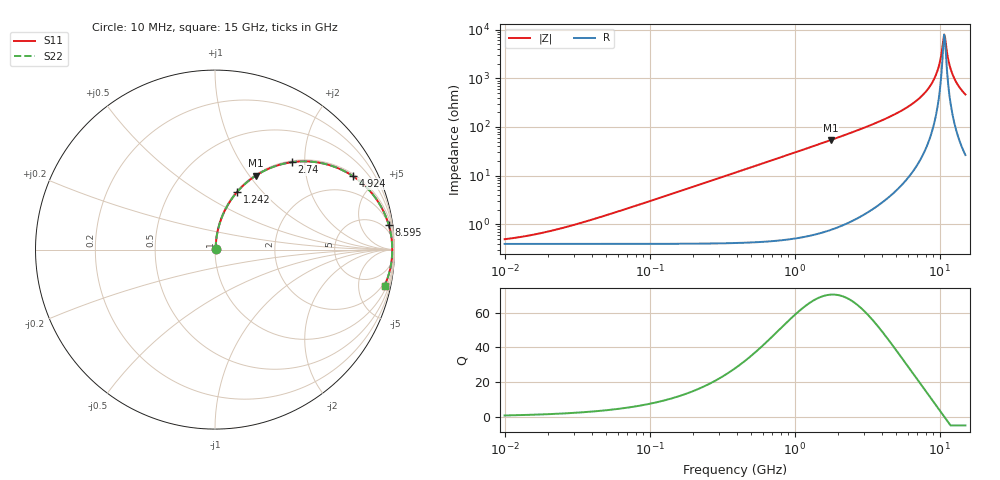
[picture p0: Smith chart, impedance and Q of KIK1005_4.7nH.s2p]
!version-3
!date-01.2023
!Series
# Hz S RI R 50
!Freq ReS11 ImS11 ReS21 ImS21 ReS12 ImS12 ReS22 ImS22
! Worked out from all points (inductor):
!   500 points, 10 MHz to 15 GHz, reference 50 ohm
!   read as one part in series: L = 4.7 nH near 40.24 MHz
!   highest Q = 70.3 at 1.765 GHz (marker M1), where L = 4.83 nH
!   self-resonance near 10.71 GHz
!   S11 on the Smith chart (normalised r, x): 10 MHz: 1.01, +0.01; 1.242 GHz: 1.01, +0.74; 2.74 GHz: 1.03, +1.73; 4.924 GHz: 1.09, +3.68; 8.595 GHz: 2, +14; 15 GHz: 1.53, -9.29
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1e7  0.00394 0.00293  0.9961 -0.00293  0.9961 -0.00293  0.00394 0.00293
1.771053e7  0.00395 0.00519  0.996 -0.00519  0.996 -0.00519  0.00395 0.00519
3.424937e7  0.00403 0.01  0.996 -0.01  0.996 -0.01  0.00403 0.01
1.155953e8  0.00509 0.0338  0.9949 -0.0338  0.9949 -0.0338  0.00509 0.0338
3.901468e8  0.0171 0.1129  0.9829 -0.1129  0.9829 -0.1129  0.0171 0.1129
1.241813e9  0.1251 0.3233  0.8749 -0.3233  0.8749 -0.3233  0.1251 0.3233
1.316788e9  0.1386 0.338  0.8614 -0.338  0.8614 -0.338  0.1386 0.338
1.765282e9  0.2263 0.4114  0.7737 -0.4114  0.7737 -0.4114  0.2263 0.4114
2.740069e9  0.4293 0.4872  0.5707 -0.4872  0.5707 -0.4872  0.4293 0.4872
4.444302e9  0.7105 0.4423  0.2895 -0.4423  0.2895 -0.4423  0.7105 0.4423
4.924452e9  0.7664 0.4105  0.2336 -0.4105  0.2336 -0.4105  0.7664 0.4105
6.89844e9  0.9132 0.2599  0.0868 -0.2599  0.0868 -0.2599  0.9132 0.2599
8.594579e9  0.9686 0.1355  0.0314 -0.1355  0.0314 -0.1355  0.9686 0.1355
9.66371e9  0.9834 0.0647  0.0166 -0.0647  0.0166 -0.0647  0.9834 0.0647
1.009808e10  0.9862 0.0378  0.0138 -0.0378  0.0138 -0.0378  0.9862 0.0378
1.055197e10  0.9876 0.0108  0.0124 -0.0108  0.0124 -0.0108  0.9876 0.0108
1.070775e10  0.9877 0.00179  0.0123 -0.00179  0.0123 -0.00179  0.9877 0.00179
1.102626e10  0.9875 -0.0162  0.0125 0.0162  0.0125 0.0162  0.9875 -0.0162
1.152187e10  0.9859 -0.0432  0.0141 0.0432  0.0141 0.0432  0.9859 -0.0432
1.22175e10  0.9814 -0.0791  0.0186 0.0791  0.0186 0.0791  0.9814 -0.0791
1.33405e10  0.9699 -0.1321  0.0301 0.1321  0.0301 0.1321  0.9699 -0.1321
1.5e10  0.9454 -0.2005  0.0546 0.2005  0.0546 0.2005  0.9454 -0.2005
